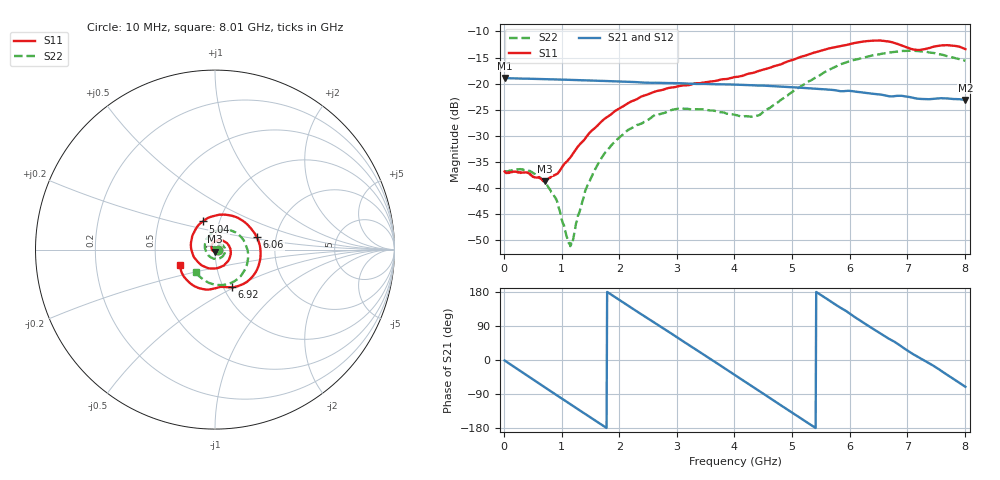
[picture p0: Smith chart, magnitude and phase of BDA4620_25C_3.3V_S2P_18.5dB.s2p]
!Agilent Technologies,E5071B,MY42404982,A.09.10
!Date: Wed May 06 08:52:39 2026
!Data & Calibration Information:
!Freq	S11:SOLT2(ON)	S21:SOLT2(ON)	S12:SOLT2(ON)	S22:SOLT2(ON)
# Hz S RI R 50
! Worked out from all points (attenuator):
!   801 points, 10 MHz to 8.01 GHz, reference 50 ohm
!   highest |S21| = -18.91 dB at 10 MHz (marker M1); lowest = -23.1 dB at 8.01 GHz (marker M2)
!   lowest |S11| = -38.7 dB at 710 MHz (marker M3), VSWR 1.02, Z = 49.7 - j1.13 ohm
!   |S11| at or under -10 dB: start of sweep to end of sweep
!   |S22| runs from -51.1 to -13.7 dB; largest |S21 - S12| = 0.00047
!   S11 on the Smith chart (normalised r, x): 10 MHz: 1.03, -0.00; 5.04 GHz: 0.83, +0.27; 6.06 GHz: 1.59, +0.23; 6.92 GHz: 1.10, -0.49; 8.01 GHz: 0.66, -0.12
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1e7  0.0144 -0.000986  0.1133 -0.00242  0.1134 -0.00243  0.0144 -0.000518
4.4e8  0.00844 -0.0109  0.0789 -0.0789  0.079 -0.079  0.0135 -0.00564
7.1e8  -0.00261 -0.0114  0.0337 -0.1054  0.0337 -0.1055  0.00829 -0.00772
9e8  -0.0112 -0.00757  -0.00265 -0.1099  -0.00281 -0.1101  0.00329 -0.00718
1.14e9  -0.0187 0.00478  -0.0468 -0.0983  -0.047 -0.0984  -0.00233 -0.00189
1.19e9  -0.0194 0.00842  -0.0551 -0.0936  -0.0553 -0.0937  -0.0031 -0.000158
1.35e9  -0.0194 0.0196  -0.0784 -0.0743  -0.0784 -0.0743  -0.00483 0.00517
1.58e9  -0.0114 0.036  -0.1002 -0.0375  -0.1002 -0.0376  -0.00402 0.0146
1.86e9  0.0104 0.05  -0.1049 0.0134  -0.105 0.0135  0.00357 0.0253
2.15e9  0.041 0.0503  -0.0843 0.0616  -0.0843 0.0617  0.0182 0.0311
2.68e9  0.0856 0.00345  -0.00324 0.1018  -0.00308 0.102  0.0468 0.0194
3.08e9  0.0771 -0.057  0.0617 0.0799  0.062 0.0798  0.0572 -0.00925
4.01e9  -0.0808 -0.0827  0.0752 -0.0628  0.0752 -0.063  -0.0133 -0.0487
4.42e9  -0.1323 0.00175  0.0156 -0.0948  0.0155 -0.0949  -0.0482 -0.0127
5.04e9  -0.0686 0.1568  -0.0735 -0.0559  -0.0737 -0.056  -0.0282 0.0813
5.35e9  0.0247 0.1943  -0.0893 -0.0101  -0.0893 -0.0102  0.0238 0.1065
6.06e9  0.2338 0.0682  -0.0375 0.0759  -0.0376 0.0761  0.1603 0.0504
6.37e9  0.2506 -0.06  0.00591 0.0803  0.00602 0.0804  0.1838 -0.0182
6.68e9  0.1815 -0.1772  0.0422 0.0631  0.0423 0.0633  0.1735 -0.0958
6.92e9  0.0954 -0.2099  0.0638 0.0421  0.0638 0.0422  0.1416 -0.1494
7.57e9  -0.0798 -0.217  0.065 -0.0324  0.0652 -0.0324  -0.0217 -0.1897
8.01e9  -0.1954 -0.088  0.023 -0.066  0.0231 -0.066  -0.1079 -0.1253
